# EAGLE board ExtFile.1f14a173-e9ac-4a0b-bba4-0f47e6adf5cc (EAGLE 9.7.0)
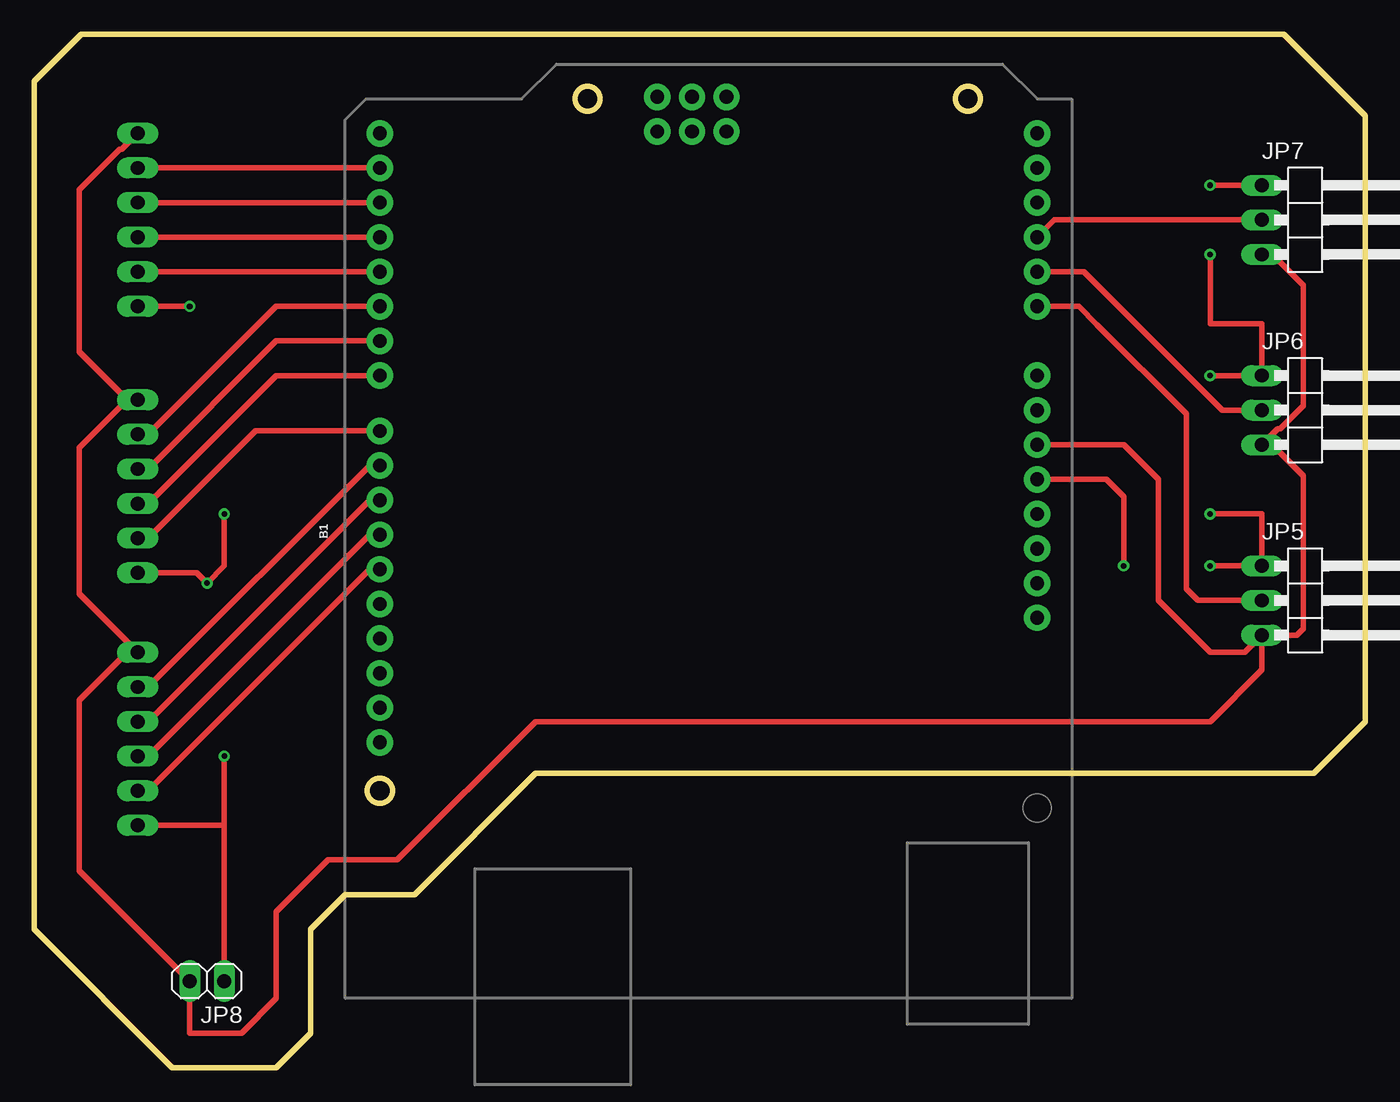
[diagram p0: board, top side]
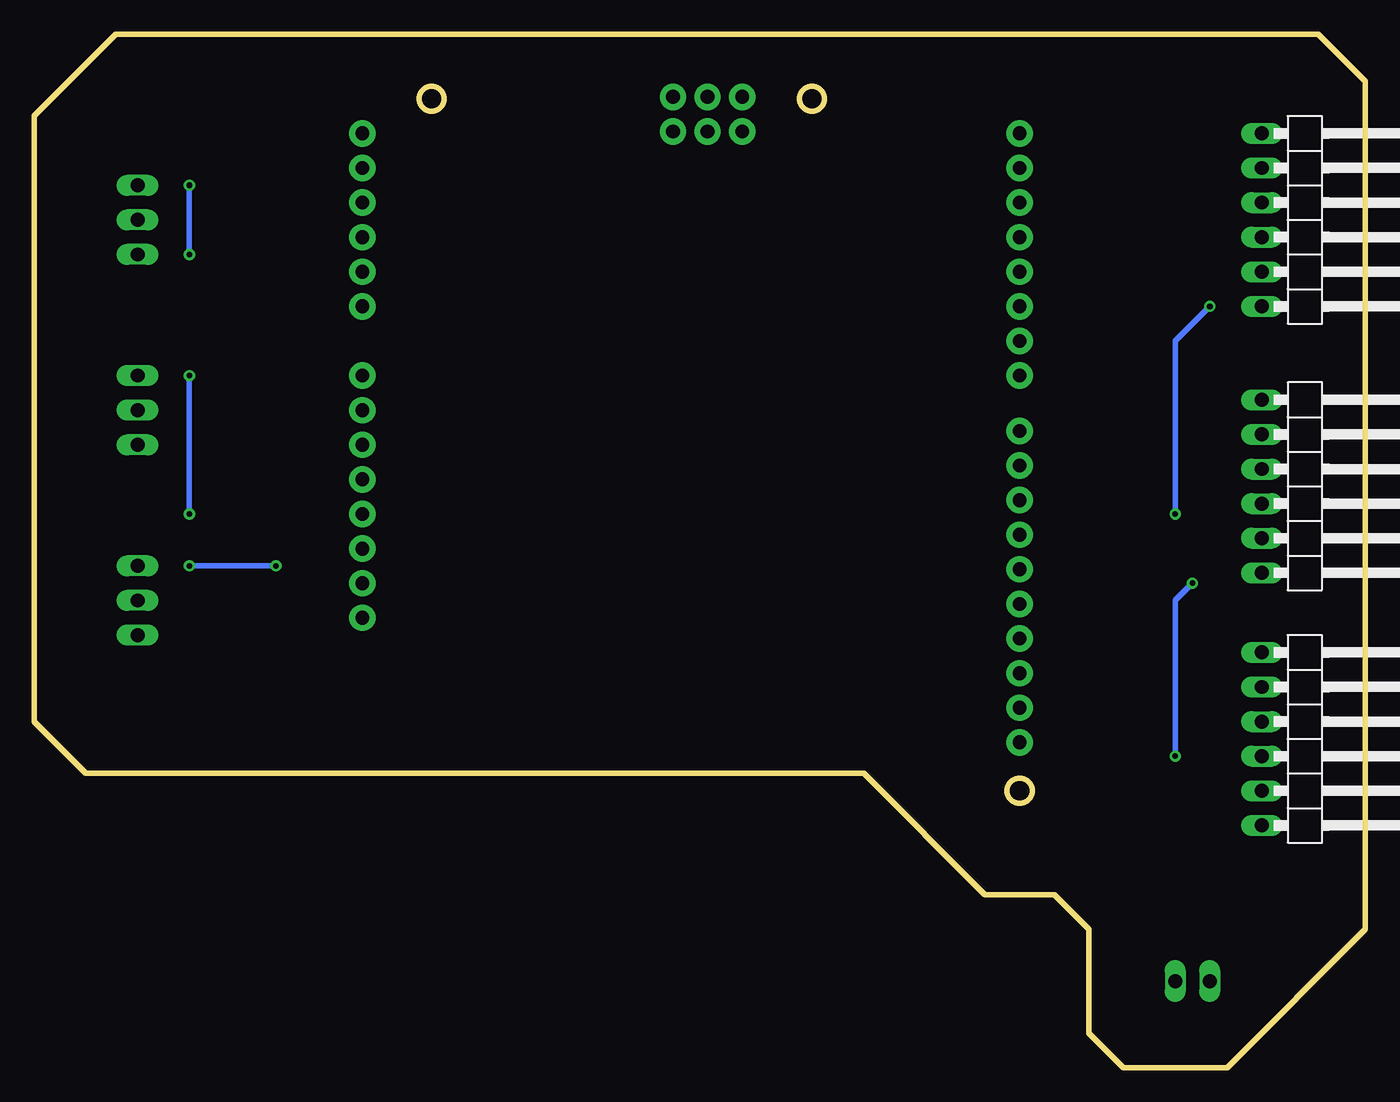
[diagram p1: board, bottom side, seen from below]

Size 97.77 x 75.87 mm. Coordinates in mm from the lower left corner, seen from the top.
Outline: 97.77,25.38 97.77,69.87 91.77,75.87 3.48,75.87 0,72.39 0,10.16 10.16,0 17.78,0 20.32,2.54 20.32,10.16 22.86,12.7 27.94,12.7 36.83,21.59 93.98,21.59 97.77,25.38
Outline: circle at 68.58,71.12 radius 0.91
Outline: circle at 40.64,71.12 radius 0.91
Outline: circle at 25.4,20.32 radius 0.91
Copper layers (1*16): Top / Bottom
Stack-up Default Layer Stack: Top User Defined 0.035mm / Dielectric-1 User Defined 1.5mm / Bottom User Defined 0.035mm
Design rules "default *": minimum track width 16mil, minimum drill 16mil, track to track 16mil, track to pad 16mil, pad to pad 16mil, via to via 16mil, smd to smd 16mil, copper to edge 40mil, drill to drill 0.25mm, minimum pad ring 10mil, minimum via ring 8mil, stop-mask expansion 4mil, vias tented up to drill 0mil, thermal gap 10mil

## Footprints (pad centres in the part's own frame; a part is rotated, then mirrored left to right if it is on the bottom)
ARDUINO_R3_NO_HOLES = drill 1.016 pad 1.93: 3.3V 1.27,-24.13; 5V 3.81,-24.13; A0 16.51,-24.13; A1 19.05,-24.13; A2 21.59,-24.13; A3 24.13,-24.13; A4 26.67,-24.13; A5 29.21,-24.13; AREF -10.414,24.13; D0 29.21,24.13; D1 26.67,24.13; D2 24.13,24.13; D3 21.59,24.13; D4 19.05,24.13; D5 16.51,24.13; D6 13.97,24.13; D7 11.43,24.13; D8 7.366,24.13; D9 4.826,24.13; D10 2.286,24.13; D11 -0.254,24.13; D12 -2.794,24.13; D13 -5.334,24.13; GND@1 6.35,-24.13; GND@2 8.89,-24.13; GND@3 -7.874,24.13; GND@4 31.89,-1.32; IOREF -3.81,-24.13; MISO 29.35,3.76; MOSI 31.89,1.22; NC -6.35,-24.13; RESET@1 -1.27,-24.13; RESET@2 29.35,-1.32; SCK 29.35,1.22; SCL -15.494,24.13; SDA -12.954,24.13; VCC 31.89,3.76; VIN 11.43,-24.13
1X06/90 = drill 1.016 long: 1 -6.35,-3.81; 2 -3.81,-3.81; 3 -1.27,-3.81; 4 1.27,-3.81; 5 3.81,-3.81; 6 6.35,-3.81
1X03/90 = drill 1.016 long: 1 -2.54,-3.81; 2 0,-3.81; 3 2.54,-3.81
1X02 = drill 1.016 long: 1 -1.27,0; 2 1.27,0

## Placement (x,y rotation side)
B1  ARDUINO_UNO_R3NO_HOLES  [ARDUINO_R3_NO_HOLES]  49.53,39.37 90 top
JP2  PINHD-1X6/90  [1X06/90]  3.81,62.23 270 bottom
JP3  PINHD-1X6/90  [1X06/90]  3.81,42.67 270 bottom
JP4  PINHD-1X6/90  [1X06/90]  3.81,24.13 270 bottom
JP5  PINHD-1X3/90  [1X03/90]  93.98,34.29 270 top
JP6  PINHD-1X3/90  [1X03/90]  93.98,48.26 270 top
JP7  PINHD-1X3/90  [1X03/90]  93.98,62.23 270 top
JP8  PINHD-1X2  [1X02]  12.7,6.35 180 top

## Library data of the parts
B1 = SparkFun-Boards
JP2-JP8 = Connector; CATEGORY: CONNECTOR; SUB-CATEGORY: PIN-HEADER

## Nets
N$1: B1.GND@1 JP2.1 JP3.1 JP4.1 JP5.3 JP6.3 JP7.3 JP8.2
N$2: JP2.6 JP3.6 JP4.6 JP8.1
N$3: B1.5V JP5.1 JP6.1 JP7.1
N$4: B1.A0 JP5.2
N$5: B1.A1 JP6.2
N$6: B1.D1 JP2.2
N$7: B1.A2 JP7.2
N$8: B1.D2 JP2.3
N$9: B1.D3 JP2.4
N$10: B1.D4 JP2.5
N$11: B1.D5 JP3.2
N$12: B1.D6 JP3.3
N$13: B1.D7 JP3.4
N$14: B1.D8 JP3.5
N$15: B1.D9 JP4.2
N$16: B1.D10 JP4.3
N$17: B1.D11 JP4.4
N$18: B1.D12 JP4.5

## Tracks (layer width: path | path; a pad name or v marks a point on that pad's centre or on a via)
N$1
  Top 0.406: 6.86,49.02 3.33,45.49 3.33,34.77 JP4.1 6.86,30.48 3.33,26.95 3.33,14.45 JP8.2 11.43,2.54 15.24,2.54 17.78,5.08 17.78,11.43 21.59,15.24 26.67,15.24 36.83,25.4 86.36,25.4 90.17,29.21 JP5.3 | JP3.1 6.86,49.02 | 6.86,49.02 3.33,52.55 3.33,64.45 6.29,67.41 6.45,67.41 JP2.1 | JP7.3 90.93,59.69 93.19,57.43 93.19,48.58 91.5,46.89 91.34,46.89 JP6.3 90.93,45.72 93.19,43.46 93.19,32.23 92.71,31.75 JP5.3 | B1.GND@1 80.01,45.72 82.55,43.18 82.55,34.29 86.36,30.48 88.9,30.48 JP5.3
N$2  (via drill 0.41 pad 0.41)
  Top 0.406: JP8.1 13.97,17.78 | 13.97,17.78 JP4.6 | JP3.6 11.94,36.32 v12.7,35.56 13.97,36.83 v13.97,40.64 | v13.97,22.86 13.97,17.78 | JP2.6 v11.43,55.88
  Bottom 0.406: v12.7,35.56 13.97,34.29 v13.97,22.86 | v11.43,55.88 13.97,53.34 v13.97,40.64
N$3  (via drill 0.41 pad 0.41)
  Top 0.406: B1.5V 78.74,43.18 80.01,41.91 v80.01,36.83 | v86.36,36.83 JP5.1 90.17,40.64 v86.36,40.64 | v86.36,50.8 JP6.1 90.17,54.61 86.36,54.61 v86.36,59.69 | v86.36,64.77 JP7.1
  Bottom 0.406: v80.01,36.83 v86.36,36.83 | v86.36,40.64 v86.36,50.8 | v86.36,59.69 v86.36,64.77
N$4
  Top 0.406: JP5.2 85.47,34.29 84.61,35.15 84.61,47.98 78.05,54.53 76.71,55.88 B1.A0
N$5
  Top 0.406: B1.A1 77.09,58.42 87.25,48.26 JP6.2
N$6
  Top 0.406: JP2.2 B1.D1
N$7
  Top 0.406: JP7.2 74.93,62.23 B1.A2
N$8
  Top 0.406: JP2.3 B1.D2
N$9
  Top 0.406: JP2.4 B1.D3
N$10
  Top 0.406: JP2.5 B1.D4
N$11
  Top 0.406: B1.D5 17.78,55.88 8.38,46.48 JP3.2
N$12
  Top 0.406: B1.D6 17.78,53.34 8.38,43.94 JP3.3
N$13
  Top 0.406: B1.D7 17.78,50.8 8.38,41.4 JP3.4
N$14
  Top 0.406: B1.D8 16.26,46.74 8.38,38.86 JP3.5
N$15
  Top 0.406: B1.D9 24.64,44.2 8.38,27.94 JP4.2
N$16
  Top 0.406: B1.D10 24.64,41.66 8.38,25.4 JP4.3
N$17
  Top 0.406: B1.D11 24.64,39.12 8.38,22.86 JP4.4
N$18
  Top 0.406: B1.D12 24.64,36.58 8.38,20.32 JP4.5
